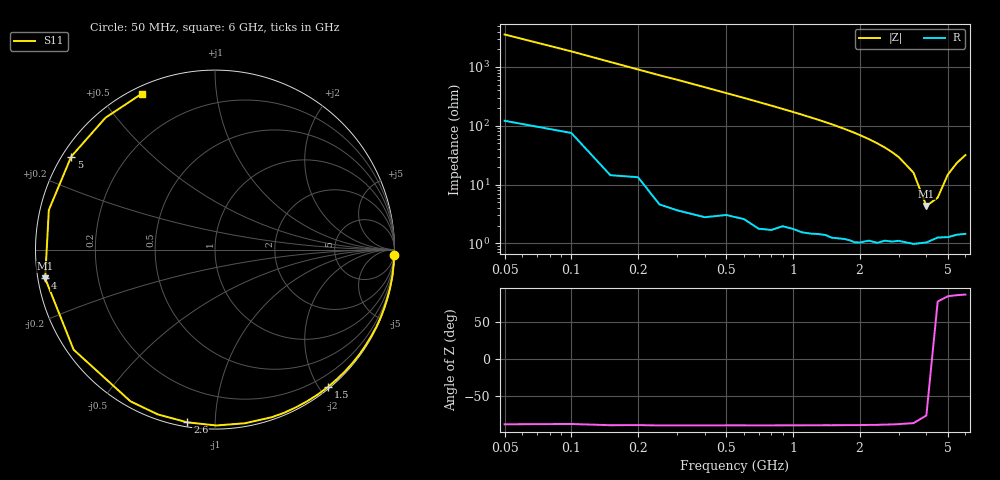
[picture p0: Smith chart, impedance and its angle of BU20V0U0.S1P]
! Infineon Technologies  Discrete & RF Semiconductors
! BB 833
! Si Tuning Diode in SOD323
! VR = 20 V
! S-Parameters:  June  1999
# GHz  S  MA  R  50
!  f  S11
! GHz  MAG  ANG
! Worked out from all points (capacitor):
!   34 points, 50 MHz to 6 GHz, reference 50 ohm
!   read as one part to ground: C = 870 fF near 50 MHz
!   lowest |Z| = 4.32 ohm at 4 GHz (marker M1)
!   series resonance near 4.208 GHz, so ESL is about 1.6 nH
!   S11 on the Smith chart (normalised r, x): 50 MHz: 2, -72; 1.5 GHz: 0.02, -2.12; 2.6 GHz: 0.02, -0.85; 4 GHz: 0.02, -0.08; 5 GHz: 0.03, +0.30; 6 GHz: 0.03, +0.63
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0.05  0.999 -1.6
0.25  0.9991 -7.9
0.4  0.9987 -12.6
0.6  0.9972 -19.0
0.7  0.9973 -22.3
0.8  0.9967 -25.6
1  0.9945 -32.4
1.1  0.9942 -35.9
1.2  0.9933 -39.5
1.3  0.9923 -43.1
1.4  0.9913 -46.8
1.5  0.9909 -50.6
1.6  0.9898 -54.6
1.7  0.9887 -58.6
1.8  0.9879 -62.7
1.9  0.9874 -66.9
2  0.986 -71.3
2.2  0.9817 -80.2
2.4  0.9799 -89.6
2.6  0.9746 -99.1
2.8  0.972 -109.1
3  0.9678 -119.1
3.5  0.9651 -144.7
4  0.9598 -170.4
4.5  0.9517 166.6
5  0.9542 147.1
5.5  0.955 129.7
6  0.9595 115.2
